ORGANIZATION_BLOCK MAIN:OB1
TITLE=Ciclo automatico A+/B+/C+/A-/B-/C
//Simulatore: 06
//Versione: 1.0
//Data: 28/02/2002
//------------- DESCRIZIONE DEL CONTROLLO ---------------------
// L'esempio utilizza tre cilindri (A, B, C) a doppio effetto e tre
// elettrovalvole 5/2 bistabili (1V1, 2V1, 3V1).
// Una valvola 3/2 monostabile 0V permette la distribuzione dell'aria al
// circuito.
// Se interviene un circuito di sicurezza esterno (simulato dal
// pulsante SB5) il PLC provvede ad azzerare l'uscita del distributore
// dell'aria (valvola 0V).
// Un Pulsante SB1 da inizio al ciclo ripetitivo che può essere
// interrotto dal pulsante di Stop SB3.
// Il pulsante SB2 da invece inizio ad un solo ciclo completo.
// Due lampade HL1, HL2 e HL3 indicano rispettivamente: la presenza
// dell'aria, il modo di funzionamento con ciclo ripetitivo e
// l'intervento del circuito di sicurezza esterna.
// I collegamenti agli ingressi del PLC sono:
// - Il selettore SA per il comando dell'aria compressa;
// - Il pulsante di arresto ciclo SB3;
// - Il pulsante di avvio ciclo in semiautomatico SB2;
// - il pulsante di avvio ciclo automatico SB1;
// - i fine corsa magnetici per il controllo della posizione
//   dei pistoni dei tre cilindri;
// - il contatto di consenso del circuito di sicurezza (simulato dal
//   pulsante SB5).
//

BEGIN
NETWORK 1 //Controllo On/Off aria compressa
//
LD I1.3 //P_SB5
A I0.6 //P_SB6
= Q0.0 //E_0Y1

NETWORK 2 //Controllo condizioni Start/Stop Ciclo
//
LD I0.7 //P_SB1
O M0.0 //Ciclo ON
A I1.1 //P_SB3
= M0.0 //Ciclo ON

NETWORK 3 //Corsa A+
//
LD M0.0 //Ciclo ON
O I1.0 //P_SB2
A I0.2 //b0
A I0.4 //c0
A I0.0 //a0
= Q0.1 //E_1Y1

NETWORK 4 //Corsa B+
//
LD I0.2 //b0
A I0.1 //a1
= Q0.3 //E_2Y1

NETWORK 5 //Corsa C+
//
LD I0.3 //b1
A I0.4 //c0
= Q0.5 //E_3Y1

NETWORK 6 //Corsa A-
//
LD I0.1 //a1
A I0.3 //b1
A I0.5 //c1
= Q0.2 //E_1Y2

NETWORK 7 //Corsa B-
//
LD I0.5 //c1
A I0.3 //b1
A I0.0 //a0
= Q0.4 //E_2Y2

NETWORK 8 //Corsa C-
//
LD I0.0 //a0
A I0.2 //b0
A I0.5 //c1
= Q0.6 //E_3Y2

NETWORK 9 //Segnalazione Presenza Aria
//
LD Q0.0 //E_0Y1
= Q0.7 //HL1

NETWORK 10 //Segnalazione Ciclo ON
//
LD M0.0 //Ciclo ON
= Q1.0 //HL2

NETWORK 11 //Segnalazione intervento sicurezza esterna
//
LDN I1.3 //P_SB5
= Q1.1 //HL3

END_ORGANIZATION_BLOCK

